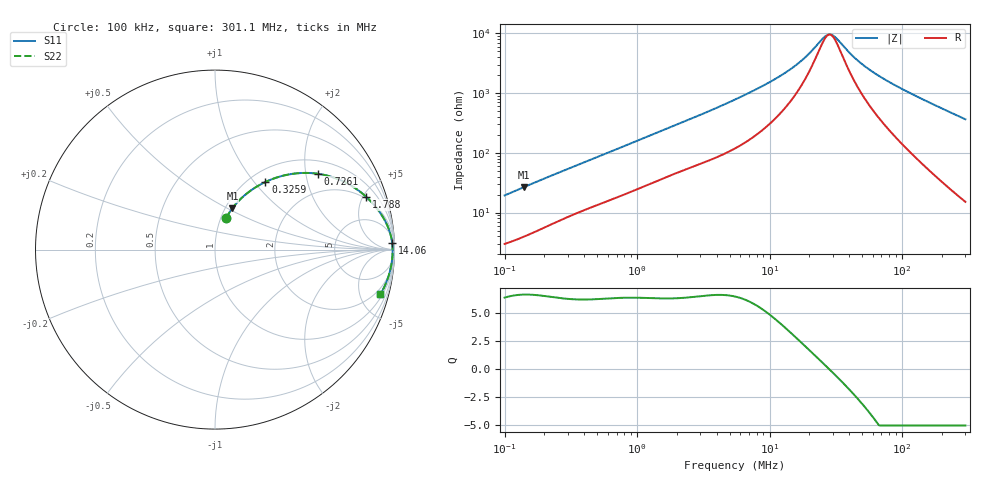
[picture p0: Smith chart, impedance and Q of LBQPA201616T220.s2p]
! LBQPA201616T220  S-PARAMETER MODEL  ( General Type )
! Model Generated by TAIYO YUDEN Corporation (http://www.ty-top.com)
! Version 1.0
! TAIYO YUDEN Control No. 191025NI43SB-FBB
! Copyright(c) 2019 TAIYO YUDEN CO.,LTD. All Rights Reserved.
! Product Description (link to TY-COMPAS)
! https://ds.yuden.co.jp/TYCOMPAS/or/detail?pn=LBQPA201616T220K&u=M
! Products Name : Inductors
! Characteristics :
!  Inductance : 22 uH , SRF(min) : 16 MHz , DC Resistance(max) : 2.34 Ohm
!  Rated Current : Saturation :250 mA , Temp Rise : 205 mA (20 degC)
!  Case Size : 2.0 x 1.6 / 0.079 x 0.063 [mm/inch] , Thickness : 1.6 / 0.063 [mm/inch]
!  (Conditions: Temperature = 25 degC , DC Bias Current/Voltage = 0A / 0V)
! External Node Assignments :
!  1  o---GGG---o  2
! GND o---------o GND
! Frequency Range : 0.1MHz  -  301.082333MHz  [ 402 STEP ]
# MHz S RI R 50
! Freq[MHz].  S11 Real  S11 Imag  S21 Real  S21 Imag  S12 Real  S12 Imag  S22 Real  S22 Imag
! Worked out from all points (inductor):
!   401 points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, 100 kHz to 301.1 MHz, reference 50 ohm
!   read as one part in series: L = 30.1 uH near 104.1 kHz
!   highest Q = 6.69 at 140.6 kHz (marker M1), where L = 30 uH
!   self-resonance near 28.39 MHz
!   S11 on the Smith chart (normalised r, x): 100 kHz: 1.06, +0.38; 325.9 kHz: 1.18, +1.14; 726.1 kHz: 1.37, +2.35; 1.788 MHz: 1.84, +5.32; 14.06 MHz: 15, +47; 301.1 MHz: 1.30, -7.30
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0.1  0.0614 0.1744  0.9386 -0.1744  0.9386 -0.1744  0.0614 0.1744
0.140554  0.0968 0.2303  0.9032 -0.2303  0.9032 -0.2303  0.0968 0.2303
0.21403  0.1701 0.3068  0.8299 -0.3068  0.8299 -0.3068  0.1701 0.3068
0.325916  0.2813 0.377  0.7187 -0.377  0.7187 -0.377  0.2813 0.377
0.382543  0.3334 0.3981  0.6666 -0.3981  0.6666 -0.3981  0.3334 0.3981
0.726064  0.5746 0.4223  0.4254 -0.4223  0.4254 -0.4223  0.5746 0.4223
1.463388  0.8 0.329  0.2 -0.329  0.2 -0.329  0.8 0.329
1.787832  0.8438 0.2927  0.1562 -0.2927  0.1562 -0.2927  0.8438 0.2927
3.009132  0.9217 0.2029  0.0783 -0.2029  0.0783 -0.2029  0.9217 0.2029
5.487097  0.9661 0.1198  0.0339 -0.1198  0.0339 -0.1198  0.9661 0.1198
9.422234  0.9822 0.067  0.0178 -0.067  0.0178 -0.067  0.9822 0.067
14.06333  0.9871 0.0385  0.0129 -0.0385  0.0129 -0.0385  0.9871 0.0385
17.52879  0.9885 0.0254  0.0115 -0.0254  0.0115 -0.0254  0.9885 0.0254
20.99048  0.9892 0.0156  0.0108 -0.0156  0.0108 -0.0156  0.9892 0.0156
26.16292  0.9896 0.00416  0.0104 -0.00416  0.0104 -0.00416  0.9896 0.00416
29.50303  0.9897 -0.00197  0.0103 0.00197  0.0103 0.00197  0.9897 -0.00197
31.96343  0.9898 -0.00606  0.0102 0.00606  0.0102 0.00606  0.9898 -0.00606
40.64564  0.9896 -0.0187  0.0104 0.0187  0.0104 0.0187  0.9896 -0.0187
48.67258  0.9891 -0.0288  0.0109 0.0288  0.0109 0.0288  0.9891 -0.0288
80.29753  0.986 -0.0629  0.014 0.0629  0.014 0.0629  0.986 -0.0629
158.6319  0.9709 -0.1353  0.0291 0.1353  0.0291 0.1353  0.9709 -0.1353
301.0823  0.9213 -0.2493  0.0787 0.2493  0.0787 0.2493  0.9213 -0.2493
